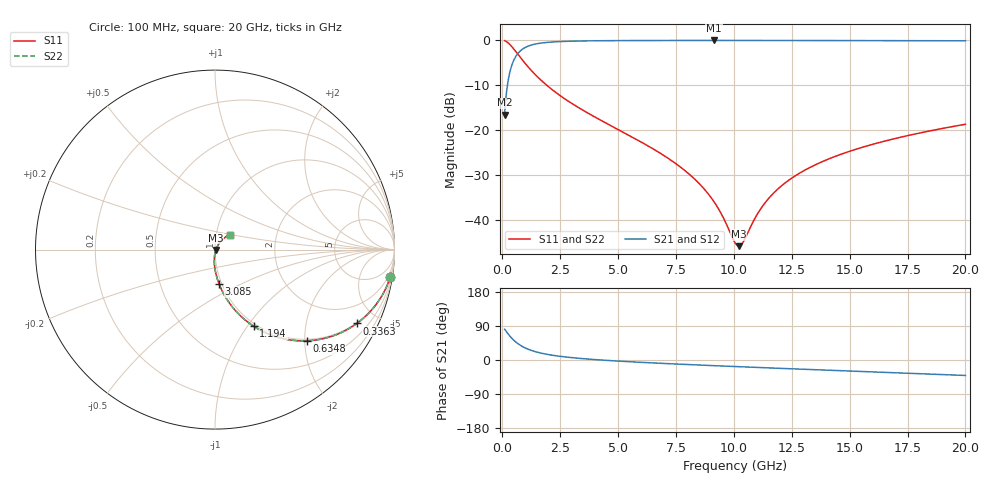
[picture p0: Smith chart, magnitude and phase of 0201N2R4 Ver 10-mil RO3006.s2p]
# GHz S MA R 50
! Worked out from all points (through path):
!   1601 points, 100 MHz to 20 GHz, reference 50 ohm
!   highest |S21| = -0.05 dB at 9.142 GHz (marker M1); lowest = -16.5 dB at 100 MHz (marker M2)
!   group delay of S21, straight-line fit = 9.55 ps
!   lowest |S11| = -45.8 dB at 10.21 GHz (marker M3), VSWR 1.01, Z = 50.5 - j0.172 ohm
!   |S11| at or under -10 dB: 1.918 GHz to end of sweep
!   |S22| runs from -45.8 to -0.1 dB; largest |S21 - S12| = 0
!   S11 on the Smith chart (normalised r, x): 100 MHz: 1, -13; 336.3 MHz: 0.97, -3.86; 634.8 MHz: 0.97, -2.04; 1.194 GHz: 0.97, -1.07; 3.085 GHz: 0.97, -0.39; 20 GHz: 1.16, +0.20
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0.1  0.9888 -8.8  0.1491 81.2  0.1491 81.2  0.9888 -8.8
0.24925  0.9357 -21.0  0.352 68.9  0.352 68.9  0.9357 -21.0
0.3363125  0.8912 -27.5  0.4525 62.4  0.4525 62.4  0.8912 -27.5
0.473125  0.8128 -36.4  0.5812 53.5  0.5812 53.5  0.8128 -36.4
0.6348125  0.7202 -44.9  0.692 45.0  0.692 45.0  0.7202 -44.9
0.896  0.591 -55.1  0.8045 34.7  0.8045 34.7  0.591 -55.1
1.1945  0.4795 -63.1  0.8751 26.6  0.8751 26.6  0.4795 -63.1
1.903437  0.3185 -74.2  0.945 15.3  0.945 15.3  0.3185 -74.2
3.085  0.1923 -83.3  0.9779 5.7  0.9779 5.7  0.1923 -83.3
3.420812  0.1704 -85.0  0.9818 3.8  0.9818 3.8  0.1704 -85.0
6.741625  0.05709 -94.0  0.9938 -8.5  0.9938 -8.5  0.05709 -94.0
8.1595  0.031 -93.7  0.9946 -12.4  0.9946 -12.4  0.031 -93.7
9.142062  0.01603 -87.1  0.9947 -15.0  0.9947 -15.0  0.01603 -87.1
10.05  0.005615 -42.0  0.9946 -17.3  0.9946 -17.3  0.005615 -42.0
10.21169  0.005132 -19.4  0.9946 -17.7  0.9946 -17.7  0.005132 -19.4
10.38581  0.005605 4.8  0.9946 -18.1  0.9946 -18.1  0.005605 4.8
11.02013  0.01172 43.5  0.9944 -19.7  0.9944 -19.7  0.01172 43.5
11.60469  0.01864 52.1  0.9942 -21.1  0.9942 -21.1  0.01864 52.1
12.37581  0.02783 55.6  0.9938 -22.9  0.9938 -22.9  0.02783 55.6
13.37081  0.0395 56.4  0.9932 -25.3  0.9932 -25.3  0.0395 56.4
16.69162  0.07761 52.3  0.9903 -33.1  0.9903 -33.1  0.07761 52.3
20  0.1164 45.8  0.9858 -40.8  0.9858 -40.8  0.1164 45.8
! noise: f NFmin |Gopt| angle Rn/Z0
0.1  0.000957  0.9556  0.5748  0.004857
2.301  0.005357  0.8259  4.3  0.006459
4.515  0.008286  0.7843  8.064  0.007855
6.729  0.01081  0.7578  11.82  0.008938
8.943  0.01312  0.7384  15.56  0.009855
11.14  0.01527  0.7235  19.24  0.01066
13.36  0.01735  0.7115  22.91  0.0114
15.57  0.01937  0.7019  26.53  0.01208
17.79  0.02135  0.6942  30.11  0.01273
20  0.0233  0.688  33.64  0.01334
